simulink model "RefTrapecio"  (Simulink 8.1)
settings: Solver=ode4  StartTime=0.0  StopTime=tmax  FixedStep=1e-3  MaxStep=1e-3  MinStep=1e-3  RelTol=1e-3
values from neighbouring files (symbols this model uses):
  kInt = 2/(-t1+t2+t3)    (= 0.00571428571429)    [RefTrapecioModeladoM.m]    (also in RefTrapecioParam.m = 2/(-t1+t2+t3))
  Km = 100    [RefTrapecioModeladoM.m]    (also in RefTrapecioM.m)
  m1 = 0.15    [RefTrapecioModeladoM.m]    (also in RefTrapecioM.m; RefTrapecioParam.m)
  m2 = 0    [RefTrapecioModeladoM.m]    (also in RefTrapecioM.m = 0.075; RefTrapecioParam.m = 0.075)
  p = 66','Color','r')    [RefTrapecioModeladoM.m]    (also in RefTrapecioM.m = 66)
  t1 = 50    [RefTrapecioModeladoM.m]    (also in RefTrapecioParam.m)
  t2 = 200    [RefTrapecioModeladoM.m]    (also in RefTrapecioM.m; RefTrapecioParam.m)
libraries: simulink x4

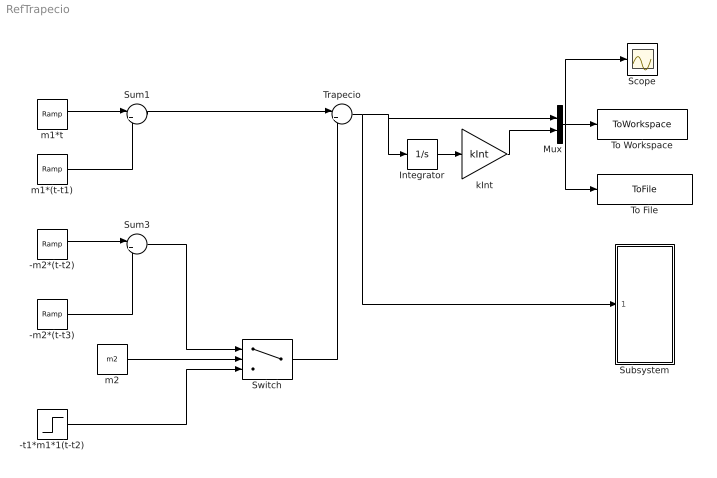
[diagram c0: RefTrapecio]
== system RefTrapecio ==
  -m2*(t-t2) : simulink/Sources/Ramp  slope=-m2  start=t2  X0=0
  -m2*(t-t3) : simulink/Sources/Ramp  slope=-m2  start=t3  X0=0
  -t1*m1*1(t-t2) : Step  Time=t2  After=-t1*m1  SampleTime=0
  Integrator : Integrator
  Mux : Mux  Inputs=2
  Scope : Scope
  Subsystem : Subsystem
  Sum1 : Sum  Inputs=|+-
  Sum3 : Sum  Inputs=|+-
  Switch : Switch  Criteria=u2 > Threshold  OutDataTypeStr=double  SampleTime=0
  To File : ToFile  Filename=TrapecioInt.mat
  To Workspace : ToWorkspace  VariableName=TrapecioInt  SampleTime=-1
  Trapecio : Sum  Inputs=|++
  kInt : Gain  Gain=kInt
  m1*(t-t1) : simulink/Sources/Ramp  slope=m1  start=t1  X0=0
  m1*t : simulink/Sources/Ramp  slope=m1  start=0  X0=0
  m2 : Constant  Value=m2
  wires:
  -m2*(t-t2)/1 -> Sum3/1
  m1*(t-t1)/1 -> Sum1/2
  Sum1/1 -> Trapecio/1
  m1*t/1 -> Sum1/1
  Trapecio/1 -> Subsystem/1(u(t)), Integrator/1, Mux/1
  Mux/1 -> Scope/1, To Workspace/1, To File/1
  Integrator/1 -> kInt/1
  kInt/1 -> Mux/2
  m2/1 -> Switch/2
  -m2*(t-t3)/1 -> Sum3/2
  Sum3/1 -> Switch/1
  Switch/1 -> Trapecio/2
  -t1*m1*1(t-t2)/1 -> Switch/3

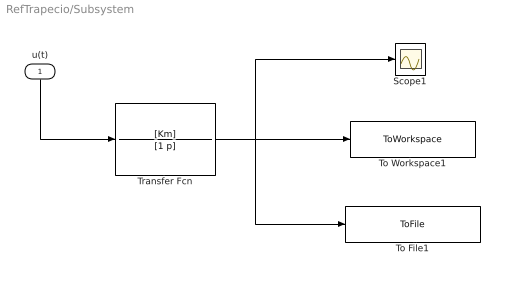
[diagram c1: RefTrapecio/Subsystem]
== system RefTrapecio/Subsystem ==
  u(t) : Inport
  Scope1 : Scope
  To File1 : ToFile  Filename=TrapecioOrdenUno.mat
  To Workspace1 : ToWorkspace  VariableName=TrapecioOrdenUno  SampleTime=-1
  Transfer Fcn : TransferFcn  Numerator=[Km]  Denominator=[1 p]
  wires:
  u(t)/1 -> Transfer Fcn/1
  Transfer Fcn/1 -> To File1/1, To Workspace1/1, Scope1/1
